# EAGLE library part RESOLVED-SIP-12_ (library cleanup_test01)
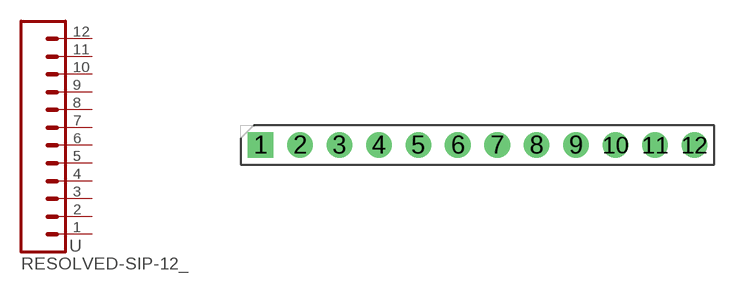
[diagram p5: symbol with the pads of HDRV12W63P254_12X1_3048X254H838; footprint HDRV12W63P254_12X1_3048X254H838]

Designator prefix -

## RESOLVED-SIP-12_2.54-SPACE-VERTICAL  [HDRV12W63P254_12X1_3048X254H838]
1  1  pas
2  2  pas
3  3  pas
4  4  pas
5  5  pas
6  6  pas
7  7  pas
8  8  pas
9  9  pas
10  10  pas
11  11  pas
12  12  pas

## Footprint HDRV12W63P254_12X1_3048X254H838 (pad centres in mm)
drill 1.1 pad 1.65 square: 1 0,0
drill 1.1 pad 1.65: 2 2.54,0; 3 5.08,0; 4 7.62,0; 5 10.16,0; 6 12.7,0; 7 15.24,0; 8 17.78,0; 9 20.32,0; 10 22.86,0; 11 25.4,0; 12 27.94,0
